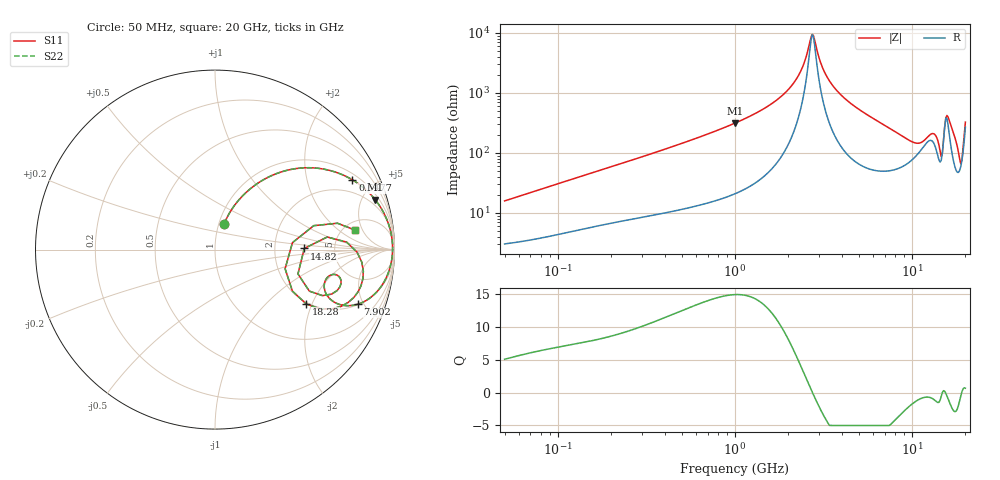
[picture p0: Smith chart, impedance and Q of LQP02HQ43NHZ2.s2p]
!Murata Part Number: LQP02HQ43NHZ2
!These Parameters are Measured in Series Mode Connection
!  o--[Z]--o
!Port1  Port2
!  o-------o
!Freq. Start=50[MHz] Stop=20[GHz], 401[Steps]
# Hz S RI R 50
!Freq.(Hz) S11(Real) S11(Imag) S21(Real) S21(Imag) S12(Real) S12(Imag) S22(Real) S22(Imag)
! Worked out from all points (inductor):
!   401 points, 50 MHz to 20 GHz, reference 50 ohm
!   read as one part in series: L = 49.3 nH near 51.52 MHz
!   highest Q = 15 at 1 GHz (marker M1), where L = 49.8 nH
!   self-resonance near 2.728 GHz
!   S11 on the Smith chart (normalised r, x): 50 MHz: 1.06, +0.31; 647.7 MHz: 1.28, +3.77; 7.902 GHz: 2.04, -4.52; 14.82 GHz: 2.98, +0.05; 18.28 GHz: 1.95, -1.82; 20 GHz: 6.37, +3.66
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5e7  0.0514 0.1435  0.9486 -0.1435  0.9486 -0.1435  0.0514 0.1435
1.364002e8  0.1741 0.3192  0.8259 -0.3192  0.8259 -0.3192  0.1741 0.3192
3.721004e8  0.5303 0.4561  0.4697 -0.4561  0.4697 -0.4561  0.5303 0.4561
6.476653e8  0.7653 0.3889  0.2347 -0.3889  0.2347 -0.3889  0.7653 0.3889
1e9  0.8925 0.2782  0.1075 -0.2782  0.1075 -0.2782  0.8925 0.2782
1.99176e9  0.9818 0.0861  0.0182 -0.0861  0.0182 -0.0861  0.9818 0.0861
2.348516e9  0.988 0.0416  0.012 -0.0416  0.012 -0.0416  0.988 0.0416
2.728004e9  0.9895 0.0012  0.0105 -0.0012  0.0105 -0.0012  0.9895 0.0012
3.168813e9  0.9869 -0.0397  0.0131 0.0397  0.0131 0.0397  0.9869 -0.0397
3.736399e9  0.9788 -0.0858  0.0212 0.0858  0.0212 0.0858  0.9788 -0.0858
7.442007e9  0.8269 -0.2918  0.1731 0.2918  0.1731 0.2918  0.8269 -0.2918
7.901521e9  0.7952 -0.3043  0.2048 0.3043  0.2048 0.3043  0.7952 -0.3043
1.019291e10  0.6275 -0.2596  0.3725 0.2596  0.3725 0.2596  0.6275 -0.2596
1.220001e10  0.6576 -0.1383  0.3424 0.1383  0.3424 0.1383  0.6576 -0.1383
1.396067e10  0.6496 -0.248  0.3504 0.248  0.3504 0.248  0.6496 -0.248
1.482269e10  0.4976 0.00658  0.5024 -0.00658  0.5024 -0.00658  0.4976 0.00658
1.527346e10  0.7333 0.0419  0.2667 -0.0419  0.2667 -0.0419  0.7333 0.0419
1.597544e10  0.8264 -0.1206  0.1736 0.1206  0.1736 0.1206  0.8264 -0.1206
1.747767e10  0.7022 -0.3165  0.2978 0.3165  0.2978 0.3165  0.7022 -0.3165
1.828096e10  0.5084 -0.303  0.4916 0.303  0.4916 0.303  0.5084 -0.303
1.88369e10  0.3905 -0.1067  0.6095 0.1067  0.6095 0.1067  0.3905 -0.1067
2e10  0.7825 0.108  0.2175 -0.108  0.2175 -0.108  0.7825 0.108
